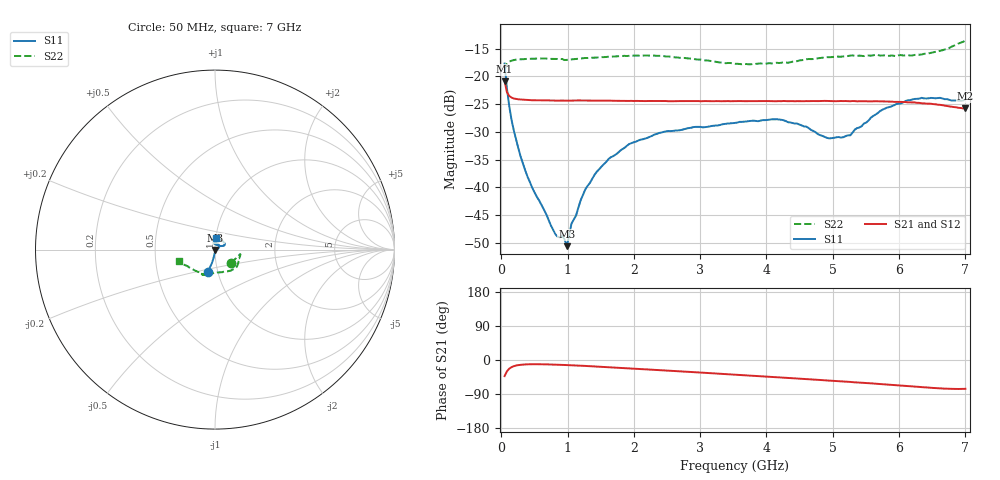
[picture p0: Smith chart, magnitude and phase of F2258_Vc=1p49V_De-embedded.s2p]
! Integrated Device Technology
! Corporate Headquarters
! 6024 Silver Creek Valley Road
! San Jose, CA 95138  USA
! Phone:  1-408-284-8200
! Toll Free:  1-800-223-1366
! Webpage:  http://www.idt.com/
! Timing and RF Division
! 515 Groton Road, Suite 102
! Westford, MA 01886-6024
! Device:  F2258
! Description: Voltage Variable RF Attenuator
! Frequency:  50.0 -  6000.00 MHz
! Package:  3x3 mm Thin QFN Plastic Package: 16 pin
! Ports:  2 RF, 2 DC
!  Pin  1  = NC
!  Pin  2  = NC
!  Pin  3  = RF2  = Port 2
!  Pin  4  = GND
!  Pin  5  = Vdd
!  Pin  6  = NC
!  Pin  7  = VCTRL
!  Pin  8  = NC
!  Pin  9  = GND
!  Pin 10  = RF1  = Port 1
!  Pin 11  = NC
!  Pin 12  = NC
!  Pin 13  = NC
!  Pin 14  = NC
!  Pin 15  = NC
!  Pin 16  = NC
! Vcntrl:  1.490 Volts
! Vdd:  +3.300 Volts
! Current:  1.161 mA
! Data:  The device was measured on a the F2258 evaluation board which has
!  individual transmission lines to the RF pins.  Data was collected
!  using a calibrated network analyzer.  The evaluation board was
!  de-embedded using a TRL calibration technique.
!  The reference plane is the edge of the package pin.
! Misc:  SN 10
!  Action Tracker AT0285
! Date Measured:  2014-12-10
! Date:  2016-01-13  MJV
! Note:
!  Integrated Device Technology supplies this data as a sample of measured
!  data at the package pin for this product.  Your particular data for this
!  product may vary.
!  Data was taken at 25 degrees C.
!  Integrated Device Technology reserves the right to change this data at anytime.
!Freq_(GHz)  S11M_(dB)  S11P_(deg)  S21M_(dB)  S21P_(deg)  S12M_(dB)  S12P_(deg)  S22M_(dB)  S22P_(deg)
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# GHz S dB R 50
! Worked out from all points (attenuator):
!   201 points, 50 MHz to 7 GHz, reference 50 ohm
!   highest |S21| = -20.86 dB at 50 MHz (marker M1); lowest = -25.8 dB at 7 GHz (marker M2)
!   lowest |S11| = -50.6 dB at 988.2 MHz (marker M3), VSWR 1.01, Z = 50.2 - j0.207 ohm
!   |S11| at or under -10 dB: start of sweep to end of sweep
!   |S22| runs from -18.9 to -13.5 dB; largest |S21 - S12| = 0.00027
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0.05  -17.66 -108.0  -20.86 -42.4  -20.87 -42.4  -18.86 -39.5
0.08475  -22.14 -102.9  -22.83 -29.9  -22.85 -29.9  -17.73 -19.9
0.15425  -27.82 -99.6  -23.81 -18.9  -23.81 -18.9  -17.16 -12.3
0.2585  -33.03 -96.8  -24.13 -13.4  -24.14 -13.4  -16.92 -10.1
0.36275  -37.00 -93.8  -24.21 -11.6  -24.23 -11.6  -16.85 -10.6
0.8145  -48.44 -40.5  -24.36 -12.2  -24.35 -12.2  -16.82 -17.4
0.91875  -48.71 -5.0  -24.35 -12.9  -24.35 -12.9  -16.85 -19.9
0.98825  -50.62 -44.5  -24.36 -13.4  -24.37 -13.4  -17.01 -20.9
1.05775  -46.57 -14.8  -24.35 -13.9  -24.36 -13.9  -16.92 -22.0
1.2315  -41.38 6.9  -24.35 -15.3  -24.36 -15.3  -16.71 -25.1
1.44  -37.20 12.1  -24.37 -17.5  -24.33 -17.5  -16.59 -28.9
1.6485  -34.60 16.8  -24.38 -19.5  -24.36 -19.5  -16.43 -32.3
1.9265  -32.21 25.7  -24.42 -22.2  -24.41 -22.2  -16.27 -36.7
2.37825  -30.21 37.4  -24.43 -26.7  -24.43 -26.7  -16.28 -44.4
3.525  -28.39 86.5  -24.45 -38.7  -24.43 -38.7  -17.70 -75.3
4.1505  -27.71 103.1  -24.47 -45.5  -24.49 -45.5  -17.52 -96.6
4.7065  -29.83 93.2  -24.43 -51.6  -24.43 -51.6  -16.86 -108.7
4.94975  -31.18 75.3  -24.45 -54.3  -24.45 -54.3  -16.52 -111.5
5.2625  -30.63 46.4  -24.47 -57.9  -24.47 -57.8  -16.23 -113.8
5.85325  -25.52 24.7  -24.53 -65.2  -24.53 -65.2  -16.28 -118.7
6.33975  -23.86 31.3  -24.84 -71.6  -24.82 -71.7  -16.04 -130.6
7  -24.09 83.5  -25.78 -76.1  -25.75 -76.1  -13.50 -162.2
